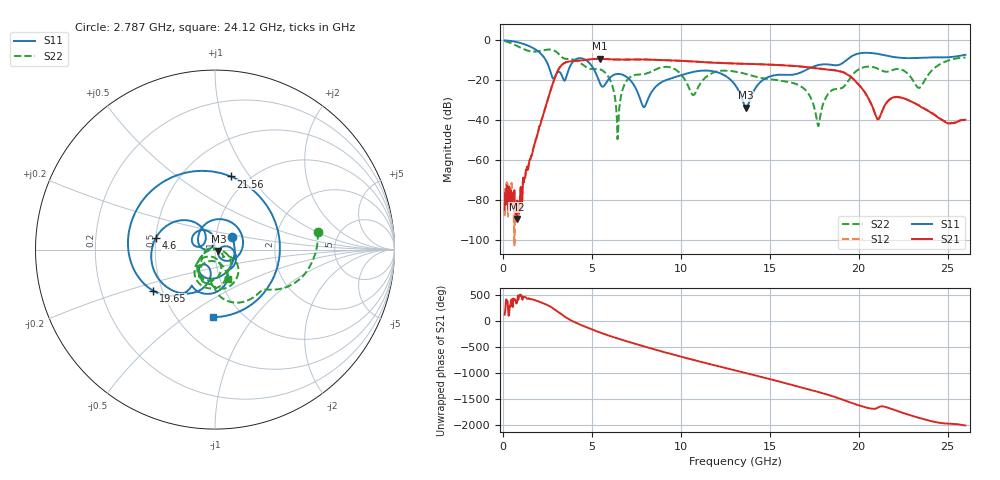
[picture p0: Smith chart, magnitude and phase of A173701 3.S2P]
!  2-Port S-parameters saved by WinCal
! VAR MeasName=S-Parameters (CALIBRATED_DATA) read from VNA (N5245A)
! VAR MeasDate=2017-6-7 10:28:38
! VAR NAME=A173701 3
! VAR FILENAME=A173701 3.S2P
! VAR DATE=2017-6-7 10:28:38
! VAR PHYS_PORTS=1,2
# Hz S DB R 50
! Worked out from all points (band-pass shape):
!   801 points, 100 MHz to 26 GHz, reference 50 ohm
!   highest |S21| = -9.17 dB at 5.442 GHz (marker M1); lowest = -89.2 dB at 779.9 MHz (marker M2)
!   |S21| within 3 dB of the highest: 3.324 GHz to 15.21 GHz (11.88 GHz wide, 128 % of centre)
!   lowest |S11| = -33.6 dB at 13.67 GHz (marker M3), VSWR 1.04, Z = 52 - j0.842 ohm
!   |S11| at or under -10 dB: 2.423 GHz to 4.012 GHz (1.589 GHz wide, 49.4 % of centre); 4.7 GHz to 19.29 GHz (14.59 GHz wide, 122 % of centre)
!   |S22| runs from -49.3 to -0.3 dB; largest |S21 - S12| = 0.0044
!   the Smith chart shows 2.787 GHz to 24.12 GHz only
!   S11 on the Smith chart (normalised r, x): 2.787 GHz: 1.19, +0.17; 4.6 GHz: 0.50, +0.07; 19.65 GHz: 0.45, -0.25; 21.56 GHz: 0.83, +0.82; 24.12 GHz: 0.74, -0.65
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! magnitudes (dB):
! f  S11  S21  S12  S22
! 100 MHz  0.0  -84.6  -87.8  -0.3
! 779.9 MHz  -0.8  -89.2  -81.5  -2.7
! 2.787 GHz  -18.6  -22.1  -22.2  -4.7
! 4.438 GHz  -9.0  -10.0  -10.0  -11.8
! 4.6 GHz  -9.5  -9.8  -9.8  -12.8
! 5.442 GHz  -21.0  -9.2  -9.2  -14.4
! 6.478 GHz  -16.7  -9.6  -9.6  -46.4
! 6.931 GHz  -18.1  -9.6  -9.6  -20.6
! 7.935 GHz  -33.4  -9.5  -9.5  -16.9
! 8.744 GHz  -21.9  -9.7  -9.8  -13.9
! 10.72 GHz  -15.7  -10.6  -10.6  -27.3
! 13.05 GHz  -22.1  -11.5  -11.5  -15.6
! 13.67 GHz  -33.6  -11.7  -11.7  -16.8
! 17.39 GHz  -13.3  -13.7  -13.6  -30.4
! 17.74 GHz  -12.3  -14.1  -14.0  -42.8
! 19.65 GHz  -7.7  -18.9  -18.9  -17.2
! 21.05 GHz  -6.7  -39.1  -39.3  -14.0
! 21.56 GHz  -7.6  -31.1  -31.4  -15.7
! 21.69 GHz  -7.8  -29.8  -30.0  -15.5
! 23.38 GHz  -8.7  -32.5  -32.4  -23.7
! 24.12 GHz  -8.5  -36.5  -36.2  -14.9
! 26 GHz  -7.2  -39.7  -39.6  -8.6
